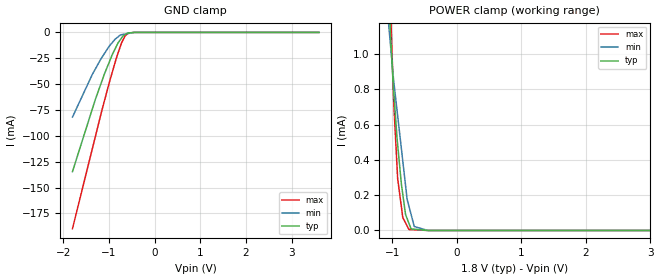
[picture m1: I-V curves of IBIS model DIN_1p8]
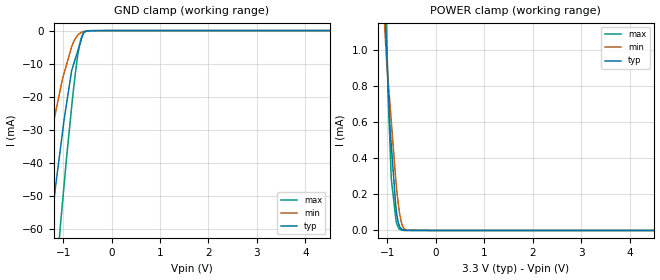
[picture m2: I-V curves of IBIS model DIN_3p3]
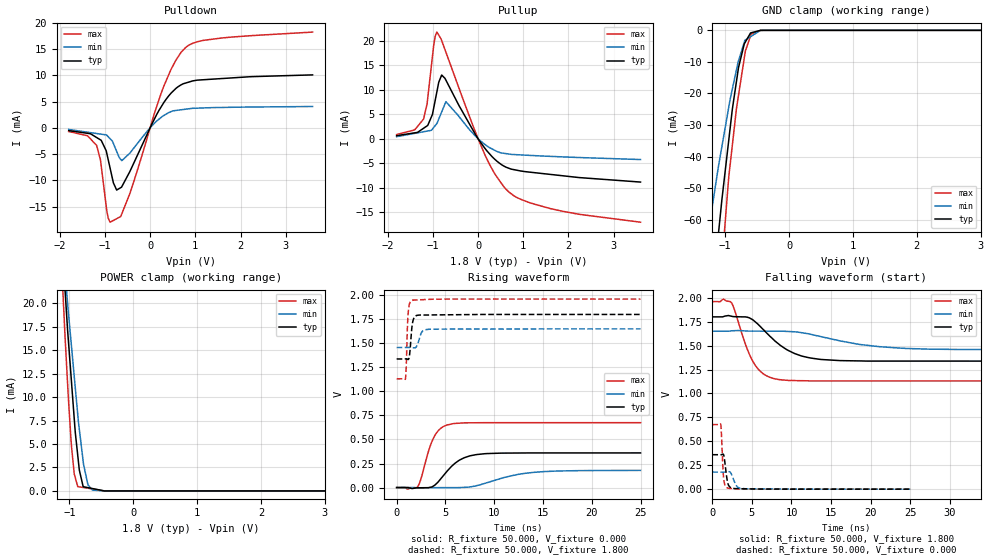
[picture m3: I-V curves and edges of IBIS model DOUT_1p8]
|Texas Instruments Incorporated
|LOW DISTORTION DIGITAL-TO-ANALOG CONVERTER FOR SEISMIC TESTING
| Marketing part#   Digital Voltage Range   Package-type   #pins
|DAC1282IPW   1.65 to 3.6   TSSOP   24
|DAC1282IPWR   1.65 to 3.6   TSSOP   24
[IBIS Ver]   4.0
[File name]   dac1282.ibs
[File Rev]   1.0
[Date]   10/12/2011
[Source]   Texas Instruments Incorporated.
   Analog-eLab, HPA
   12500 TI Blvd
   Dallas, TX -75243
   For Support e-mail: elab_ibis@list.ti.com
[Notes]   Revision History:
   1.0: 10/12/2011
   - Initial version of the model
   - Initial Model generated from simulations in TISPICED
   - Model names with a trailing _1p8 contains the model for
   1.8V (1.65V and 1.96V).
   _ Model names with trailing _3p3 contains
   the model for 3.3V (3V and 3.6V) operation.
   - Model not matched to measurements
   - C_comp although listed in numerical order of value are
   obtained from varying PVT conditions. For PVT conditions
   for each specific value refer the buffer description under
   respective [Model]. IBIS model user is responsible for using
   appropriate C_comp to simulate for Signal Integrity.
   - Combined Pulldown non-monotonic warnings for DOUT_1p8 and
   DOUT_3p3 maximum errors are minimal and
   based on SPICE simulations.
[Disclaimer]
  This model is designed as an aid for customers of Texas Instruments.
  TI and its licensors and suppliers make no warranties, either expressed
  or implied, with respect to this model, including the warranties of
  merchantability or fitness for a particular purpose.  The model is
  provided solely on an "as is" basis.  The entire risk as to its quality
  and performance is with the customer.
[Copyright] (C) Copyright 2011 Texas Instruments Incorporated.
   All rights reserved.
|   DAC1282
[Component]   dac1282pw
[Manufacturer] TI
[Package]   | 24 TSSOP - PW package
| variable   typ   min   max
R_pkg  0.104   0.026   0.213
L_pkg  2.117nH  1.475nH  3.401nH
C_pkg  0.480pF  0.412pF  0.691pF
|-------------------------PIN------------------------------------------------
[Pin] signal_name  model_name  R_pin  L_pin C_pin
1   _CS   DIN   0.02588  1.99587nH  0.69055pF
2   SCLK   DIN   0.18891  2.89647nH  0.54679pF
3   DIN   DIN   0.14483  2.02547nH  0.41167pF
4   DOUT   DOUT   0.17891  2.31159nH  0.43773pF
5   DVDD   POWER   0.07668  1.70928nH  0.46198pF
6   DGND   GND   0.06729  1.57986nH  0.45212pF
7   CLK   DIN   0.12296  1.83443nH  0.41811pF
8   SW/TD   DIN   0.14416  2.01514nH  0.42683pF
9   SYNC   DIN   0.18683  2.38497nH  0.44048pF
10  _RESET/_PWDN  DIN   0.14483  2.02654nH  0.41150pF
11  DGND   GND   0.18893  2.90636nH  0.54252pF
12  VREF   TERM   0.21309  3.40115nH  0.59253pF
13  AVDD   POWER   0.06979  2.67428nH  0.65001pF
14  AVSS   GND   0.09591  2.42393nH  0.59072pF
15  CAPN   TERM   0.06130  1.96860nH  0.48443pF
16  VOUTN   TERM   0.05220  1.71081nH  0.47339pF
17  SWINN   TERM   0.04793  1.57518nH  0.47031pF
18  SWOUTN   TERM   0.04349  1.47845nH  0.46682pF
19  SWOUTP   TERM   0.04349  1.47490nH  0.46677pF
30  SWINP   TERM   0.04793  1.56459nH  0.47033pF
21  VOUTP   TERM   0.05169  1.71740nH  0.47001pF
22  CAPP   TERM   0.06171  1.96903nH  0.47638pF
23  AVSS   POWER   0.09587  2.41513nH  0.58921pF
24  AVDD   GND   0.06960  2.63357nH  0.63953pF
|   Model Selectors
[Model Selector]  DIN
DIN_1p8   1.8 V digital input
DIN_3p3   3.3 V digital input
|NOTES   Model DIN split into two Models DIN_1p8 and DIN_3p3
|   to accomodate vast voltage range of 1.65 V - 3.6V
|   DIN_1p8 operates in voltage range of 1.65 - 1.8 - 1.96
|   DIN_3p3 operates in voltage range of 3 - 3.3 - 3.6
|   The max pin frequency for Model DIN is 8.8 MHz.Also the
|   voltage range and frequency is referenced with datasheet.
[Model Selector]  DOUT
DOUT_1p8   1.8 V digital output
DOUT_3p3   3.3 V digital output
|NOTES   Model DOUT split into two Models DOUT_1p8 and DOUT_3p3
|   to accomodate vast voltage range of 1.65 V - 3.6V
|   DOUT_1p8 operates in voltage range of 1.65 - 1.8 - 1.96
|   DOUT_3p3 operates in voltage range of 3 - 3.3 - 3.6
|   The max pin frequency for Model DOUT is 8.8 MHz.Also the
|   voltage range and frequency is referenced with datasheet.
[Model Selector]  TERM
TERM_1p8   1.8 V digital output
TERM_3p3   3.3 V digital output
|   TERM Model
[Model] TERM_1p8
Model_type Terminator
C_comp   1e-20   1e-20   1e-20
| variable   typ   min   max
[Voltage Range]   1.8V   1.65V   1.96V
[POWER Clamp Reference]  1.8V   1.65V   1.96V
[GND Clamp Reference]   0.0V   0.0V   0.0V
|Operating Temperature   27   85   -40
[Temperature Range]   30   88   -40
[Model] TERM_3p3
Model_type Terminator
C_comp   1e-20   1e-20   1e-20
| variable   typ   min   max
[Voltage Range]   3.3V   3.0V   3.6V
[POWER Clamp Reference]  3.3V   3.0V   3.6V
[GND Clamp Reference]   0.0V   0.0V   0.0V
|Operating Temperature   27   85   -40
[Temperature Range]   30   88   -40
| Models and submodels in the file (6): DIN_1p8 (Input), DIN_3p3 (Input), DOUT_1p8 (3-state), DOUT_3p3 (3-state), TERM_1p8 (Terminator), TERM_3p3 (Terminator)
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|NOTES   Model TERM split into two Models TERM_1p8 and TERM_3p3
|   to accomodate vast voltage range of 1.65 V - 3.6V
|   TERM_1p8 operates in voltage range of 1.65 - 1.8 - 1.96
|   TERM_3p3 operates in voltage range of 3 - 3.3 - 3.6
|   DIN Model
[Model] DIN_1p8
Model_type   Input
Vinl = 0.36
Vinh = 1.44
|   typ   min   max
|   (nom PVT)   (Fast PVT)   (slow PVT)
C_comp   1.770E-12   1.426E-12   2.090E-12
| Where   nom PVT is  Nominal Process, 1.8V, 30C
|   Fast PVT is Strong Process, 1.96V, -40C
|   Slow PVT is Weak Process, 1.65V, 88C
|C_comp - from L-C Tank method, L = 1nH, peak frequency
[Model Spec]   |1.8 V
Vinl  0.36 0.33 0.392
Vinh  1.44 1.32 1.568
|Vinl = 0.2 DVDD
|Vinh = 0.8 DVDD
[Voltage Range]   1.8   1.65   1.96
[Temperature Range]   30   88   -40
[Power Clamp Reference]   1.8   1.65   1.96
[GND Clamp Reference]   0   0   0
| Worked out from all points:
|   GND clamp passes 1 mA (typ) near -0.61 V on its own axis
|   POWER clamp passes 1 mA (typ) near -1.01 V on its own axis
[GND Clamp]
|   Voltage   I(typ)   I(min)   I(max)
-1.8V     -134.6mA   -81.87mA   -189.7mA
-1.368V   -74.4mA    -40.88mA   -113mA
-1.294V   -64.11mA   -34.93mA   -99.8mA
-1.101V   -40.27mA   -20.49mA   -66.29mA
-931.1mV  -21.74mA   -9.988mA   -38.82mA
-821.8mV  -11.96mA   -4.985mA   -22.41mA
-723.4mV  -5.25mA    -2.186mA   -9.925mA
-692.4mV  -3.372mA   -1.941mA   -7.247mA
-643.9mV  -1.994mA   -1.558mA   -3.151mA
-572mV    -553.2uA   -990.5uA   -639.6uA
-444.4mV  -15uA      -14.68uA   -13.36uA
3.595V    0A         0A         0A
[POWER Clamp]
|   Voltage   I(typ)   I(min)   I(max)
-1.8V     10.46mA    8.161mA    13.21mA
-1.072V   1.48mA     1.235mA    1.832mA
-1.028V   1.109mA    1.053mA    1.267mA
-983.8mV  816.4uA    871.1uA    785.3uA
-916.7mV  486.5uA    650.9uA    294.5uA
-837.7mV  206.6uA    395.8uA    75.69uA
-793.4mV  89.78uA    252.6uA    42.31uA
-768.2mV  65.68uA    174.5uA    24.46uA
-741.3mV  40.01uA    136.9uA    5.45uA
-659.6mV  7.323uA    22.63uA    3.951uA
-448.7mV  0A         24.73nA    80.01nA
3.595V    0A         0A         0A
[Model] DIN_3p3
Model_type   Input
Vinl = 0.66
Vinh = 2.64
|   typ   min   max
|   (nom PVT)   (Fast PVT)   (slow PVT)
C_comp   1.637E-12   1.343E-12   1.959E-12
| Where   nom PVT is  Nominal Process, 3.3V, 30C
|   Fast PVT is Strong Process, 3.6V, -40C
|   Slow PVT is Weak Process, 3.0V, 88C
|C_comp - from L-C Tank method, L = 1nH, peak frequency
[Model Spec]   |3.3 V
Vinl  0.66 0.6 0.72
Vinh  2.64 2.4 2.88
|Vinl = 0.2 DVDD
|Vinh = 0.8 DVDD
[Voltage Range]   3.3   3   3.6
[Temperature Range]   30   88   -40
[Power Clamp Reference]   3.3   3   3.6
[GND Clamp Reference]   0   0   0
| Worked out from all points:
|   GND clamp passes 1 mA (typ) near -0.59 V on its own axis
|   POWER clamp passes 1 mA (typ) near -1.02 V on its own axis
[GND Clamp]
|   Voltage   I(typ)   I(min)   I(max)
-3.3V     -363.8mA   -257.2mA   -460.2mA
-1.598V   -105.6mA   -62.12mA   -153.8mA
-1.344V   -70.8mA    -39.22mA   -108.1mA
-1.245V   -58.18mA   -30.83mA   -91.14mA
-1.157V   -46.86mA   -24.54mA   -75.87mA
-1.043V   -33.92mA   -16.56mA   -56.36mA
-825mV    -12mA      -4.861mA   -22.88mA
-772.6mV  -9.549mA   -3.08mA    -15.79mA
-665.4mV  -4.547mA   -925.3uA   -4.549mA
-599.3mV  -1.467mA   -344.1uA   -1.249mA
-18.32mV  0A         0A         0A
6.59V     0A         0A         0A
[POWER Clamp]
|   Voltage   I(typ)   I(min)   I(max)
-3.3V     30.76mA    25.53mA    38.05mA
-1.093V   1.648mA    1.305mA    2.053mA
-1.042V   1.16mA     1.065mA    1.433mA
-1.013V   979.4uA    928uA      1.081mA
-984.4mV  798.2uA    827.7uA    745.7uA
-948.9mV  576uA      704.7uA    492.7uA
-919.8mV  470.7uA    603.6uA    284.7uA
-825mV    128.1uA    274.6uA    64.82uA
-770.9mV  39.93uA    138.1uA    15.68uA
-722.2mV  12.06uA    57.51uA    2.817uA
-597mV    740.2nA    1.805uA    74.47nA
6.59V     0A         0A         0A
|   DOUT Model
[Model] DOUT_1p8
Model_type   3-state
Polarity   Inverting
Vmeas = 0.7
Vref = 0.7
Cref = 2pF
Rref = 50
|   typ   min   max
|   (nom PVT)   (Fast PVT)   (slow PVT)
|   BUFFER OUTPUT TURNED HIGH
C_comp   2.466E-12   1.862E-12   3.105E-12
|   BUFFER OUTPUT LOW
|C_comp   3.105E-12   1.941E-12   3.222E-12
|   BUFFER HIGH Z STATE
|C_comp   3.222E-12   1.854E-12   3.119E-12
| Where   nom PVT is  Nominal Process, 1.8V, 30C
|   Fast PVT is Strong Process, 1.96V, -40C
|   Slow PVT is Weak Process, 1.65V, 88C
|C_comp - from L-C Tank method, L = 1nH, peak frequency
[Voltage Range]   1.8   1.65   1.96
[Temperature Range]   30   88   -40
[Pullup Reference]   1.8   1.65   1.96
[Pulldown Reference]   0   0   0
[Power Clamp Reference]   1.8   1.65   1.96
[GND Clamp Reference]   0   0   0
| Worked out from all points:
|   slope of the pulldown table from 0 to 0.27 V, typ, clamps not added: 62 ohm
|   slope of the pullup table from 0 to 0.27 V, typ, clamps not added: 83 ohm
|   GND clamp passes 1 mA (typ) near -0.61 V on its own axis
|   POWER clamp passes 1 mA (typ) near -0.80 V on its own axis
|   falling waveform, R_fixture 50.000, V_fixture 1.800: 20-80 % time 4.12ns typ, 7.65ns min, 2.31ns max; typ from 1.8 V to 1.34 V
|   rising waveform, R_fixture 50.000, V_fixture 0.000: 20-80 % time 2.12ns typ, 4.03ns min, 1.29ns max; typ from 0 V to 0.36 V
|   rising waveform, R_fixture 50.000, V_fixture 1.800: 20-80 % time 247ps typ, 383ps min, 173ps max; typ from 1.34 V to 1.8 V
|   falling waveform, R_fixture 50.000, V_fixture 0.000: 20-80 % time 355ps typ, 560ps min, 232ps max; typ from 0.36 V to 0 V
[Pulldown]
|   Voltage   I(typ)   I(min)   I(max)
-1.8V     -525.9uA   -305.7uA   -688uA
-1.384V   -1.039mA   -826.6uA   -1.511mA
-1.185V   -1.83mA    -1.076mA   -3.323mA
-1.098V   -2.288mA   -1.185mA   -6.099mA
-971.7mV  -4.35mA    -1.343mA   -14.87mA
-884.4mV  -7.691mA   -2.068mA   -17.98mA
-740.3mV  -11.84mA   -4.466mA   -17.32mA
-631.5mV  -11.3mA    -6.2mA     -16.5mA
303.5mV   4.822mA    2.355mA    7.949mA
790.2mV   8.553mA    3.56mA     15.35mA
1.592V    9.402mA    3.889mA    17.14mA
3.595V    10.1mA     4.069mA    18.25mA
[GND Clamp]
|   Voltage   I(typ)   I(min)   I(max)
-1.8V     -213.5mA   -143.4mA   -305.2mA
-1.251V   -93.42mA   -62.37mA   -133.5mA
-1.107V   -64.84mA   -43.38mA   -90.53mA
-1.05V    -53.57mA   -36.77mA   -73.93mA
-946.3mV  -35.32mA   -24.67mA   -47.18mA
-891mV    -25.61mA   -18.96mA   -37.05mA
-822.5mV  -16.14mA   -12.49mA   -24.75mA
-790.7mV  -11.8mA    -9.667mA   -20.59mA
-684.8mV  -3.749mA   -3.078mA   -6.75mA
-602.2mV  -827.3uA   -2.011mA   -1.785mA
-447.8mV  -18.38uA   -17.75uA   -28.96uA
3.595V    0A         0A         0A
[Pullup]
|   Voltage   I(typ)   I(min)   I(max)
-1.8V     601.2uA    401.5uA    830.5uA
-1.4V     1.185mA    1.077mA    1.798mA
-1.206V   2.103mA    1.403mA    3.968mA
-1.124V   2.618mA    1.542mA    7.273mA
-1.009V   4.92mA     1.946mA    16.68mA
-909.3mV  9.586mA    3.094mA    21.74mA
-805.3mV  12.95mA    5.411mA    20.05mA
-710.4mV  11.94mA    7.544mA    17.65mA
153.5mV   -1.989mA   -1.191mA   -3.315mA
677.7mV   -6.028mA   -3.134mA   -10.84mA
1.592V    -7.291mA   -3.612mA   -14.25mA
3.595V    -8.862mA   -4.265mA   -17.05mA
[POWER Clamp]
|   Voltage   I(typ)   I(min)   I(max)
-1.8V     105.9mA    90.04mA    127.6mA
-1.185V   34.01mA    33.21mA    33.2mA
-1.064V   21.07mA    23.09mA    16.06mA
-1.027V   17.19mA    20.04mA    11.48mA
-966.6mV  11.68mA    15.47mA    4.82mA
-923.1mV  7.73mA     12.24mA    1.816mA
-867.5mV  3.768mA    8.117mA    459.2uA
-843.1mV  2.219mA    6.565mA    432.6uA
-777.7mV  443.4uA    2.863mA    361.3uA
-710.4mV  352.3uA    714uA      288uA
-639mV    255.6uA    92.05uA    210.1uA
3.595V    0A         0A         0A
[Ramp]
R_load = 50
|   typ   min   max
dV/dt_r   0.216099/2.11423e-009   0.10702/4.00133e-009  0.404832/1.29059e-009
dV/dt_f   0.280937/4.08061e-009  0.116178/7.43517e-009  0.497718/2.30207e-009
[Falling Waveform]
R_fixture = 50.000
V_fixture = 1.800
V_fixture_min = 1.650
V_fixture_max = 1.960
C_fixture = 0.000
|  time   V(typ)   V(min)   V(max)
0s        1.8V       1.65V      1.96V
2.414ns   1.807V     1.654V     1.948V
4.231ns   1.799V     1.653V     1.502V
5.238ns   1.761V     1.651V     1.318V
6.368ns   1.673V     1.65V      1.209V
8.002ns   1.542V     1.65V      1.151V
11.24ns   1.392V     1.635V     1.133V
16.14ns   1.343V     1.549V     1.131V
24.45ns   1.338V     1.47V      1.131V
50ns      1.337V     1.456V     1.13V
[Rising Waveform]
R_fixture = 50.000
V_fixture = 0.000
V_fixture_min = 0.000
V_fixture_max = 0.000
C_fixture = 0.000
|  time   V(typ)   V(min)   V(max)
0s        48.67nV    135.1nV    44.05nV
2.143ns   -2.651mV   -2.397mV   8.103mV
2.501ns   -2.23mV    -5.141mV   93.27mV
3.758ns   15.25mV    -1.13mV    510.6mV
4.305ns   64.36mV    -1.012mV   595.3mV
5.179ns   171.2mV    -822.2uV   651.1mV
6.919ns   309.6mV    1.892mV    672.4mV
9.03ns    351.8mV    43.16mV    674.5mV
14.01ns   359.8mV    157.6mV    674.5mV
25ns      360.2mV    178.4mV    674.7mV
[Rising Waveform]
R_fixture = 50.000
V_fixture = 1.800
V_fixture_min = 1.650
V_fixture_max = 1.960
C_fixture = 0.000
|  time   V(typ)   V(min)   V(max)
0s        1.337V     1.456V     1.13V
903.5ps   1.338V     1.457V     1.132V
982.5ps   1.338V     1.457V     1.256V
1.118ns   1.334V     1.457V     1.701V
1.204ns   1.333V     1.457V     1.838V
1.341ns   1.394V     1.457V     1.918V
1.667ns   1.731V     1.454V     1.949V
2.617ns   1.794V     1.623V     1.953V
3.362ns   1.794V     1.647V     1.957V
25ns      1.8V       1.65V      1.96V
[Falling Waveform]
R_fixture = 50.000
V_fixture = 0.000
V_fixture_min = 0.000
V_fixture_max = 0.000
C_fixture = 0.000
|  time   V(typ)   V(min)   V(max)
0s        360.2mV    178.4mV    674.7mV
1.056ns   359.7mV    178.1mV    678.4mV
1.149ns   360.1mV    178.1mV    575.4mV
1.344ns   366.4mV    178mV      203.1mV
1.442ns   353.7mV    178mV      101.8mV
1.896ns   83.07mV    181.1mV    13.69mV
2.071ns   37.21mV    182.9mV    8.916mV
3.152ns   5.293mV    23.65mV    3.171mV
4.238ns   3.67mV     3.567mV    1.562mV
25ns      1.16nV     115.7nV    1.017nV
